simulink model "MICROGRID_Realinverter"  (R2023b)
settings: Solver=ode23tb  StartTime=0  StopTime=1.5  FixedStep=1e-3  RelTol=1e-5
undefined symbols (not defined in the file or in its folder): bridge, phase, pulses, Three
libraries: spsThreePhaseSeriesRLCBranchLib x11, simulink x10, spsThreePhaseVIMeasurementLib x9, slpidlib x8, spsMeanLib x8, spsabctodq0Lib x5, spsPLL3phLib x5, spsPower3phInstantaneousLib x5, spsRMSLib x5, spsCurrentMeasurementLib x4, spsDCVoltageSourceLib x4, spsPWMGenerator2LevelLib x4
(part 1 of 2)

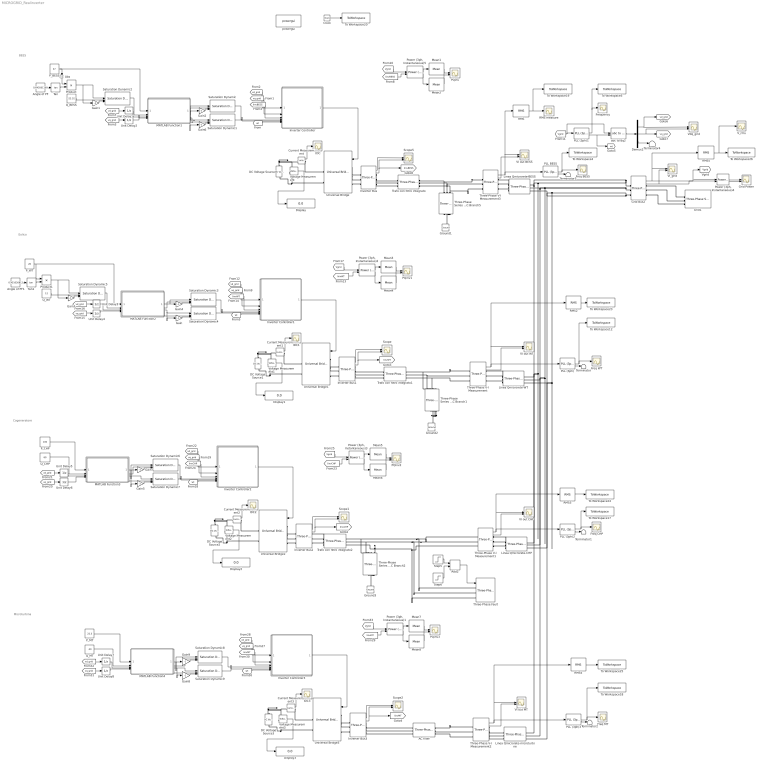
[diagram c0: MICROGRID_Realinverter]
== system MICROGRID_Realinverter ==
  note: BEES
  note: Eolico
  note: Cogeneratore
  note: Microturbina
  AC filter : spsThreePhaseSeriesRLCBranchLib/Three-Phase Series RLC Branch  LConnTagsString=A|B|C  RConnTagsString=A|B|C  BranchType=L  Resistance=0.017887  Inductance=0.536e-3  Capacitance=1e-6  Measurements=None
  Abs : Abs
  Add2 : Sum
  Angle of PF : Constant  Value=0.643501109
  Angle of PF1 : Constant  Value=0.451026812
  Clock : Clock
  Current Measurement{,1..3} (4 alike) : spsCurrentMeasurementLib/Current Measurement  PhasorSimulation=off  OutputType=Complex  PSBequivalent=0
  DC Voltage Source : spsDCVoltageSourceLib/DC Voltage Source  Amplitude=620  Measurements=None
  DC Voltage Source1 : spsDCVoltageSourceLib/DC Voltage Source  Amplitude=800  Measurements=None
  DC Voltage Source2 : spsDCVoltageSourceLib/DC Voltage Source  Amplitude=620  Measurements=None
  DC Voltage Source3 : spsDCVoltageSourceLib/DC Voltage Source  Amplitude=760  Measurements=None
  Demux2 : Demux  Outputs=3
  Display{,1..3} (4 alike) : Display
  Freq BESS : Scope
  Freq CHP : Scope
  Freq MT : Scope
  Freq WT : Scope
  Frequency : Scope
  Gain{,1..9} (10 alike) : Gain  Gain=-1
  Grid Bus2 : spsThreePhaseVIMeasurementLib/Three-Phase V-I Measurement  VoltageMeasurement=phase-to-ground  SetLabelV=off  LabelV=Vabc  Vpu=off  VpuLL=off  CurrentMeasurement=yes  SetLabelI=off  LabelI=Iabc  Ipu=off  Pbase=100e6  Vbase=500e3  OutputType=Complex  PhasorSimulation=off  PSBequivalent=0
  Grid Power : Scope  NumInputPorts=2
  Grid1 : spsThreePhaseSourceLib/Three-Phase Source  InternalConnection=Yg  VoltagePhases=off  Voltage=400  PhaseAngle=0  Voltage_phases=[25e3 25e3 25e3]/sqrt(3)  PhaseAngles_phases=[0 -120 +120]  Frequency=50  NonIdealSource=on  SpecifyImpedance=off  Resistance=86.7007e-4  Inductance=5.7558e-5  ShortCircuitLevel=100e6  BaseVoltage=400  XRratio=7  BusType=swing  Pref=10e3  Qref=0  Prefabc=[10e3, 10e3, 10e3]  Qrefabc=[0, 0, 0]  Qmin=-inf  Qmax=inf
  Ground1 : spsGroundLib/Ground  LConnTagsString=a
  Ground2 : spsGroundLib/Ground  LConnTagsString=a
  Ground3 : spsGroundLib/Ground  LConnTagsString=a
  IDC{,1..3} (4 alike) : Scope
  Inverter Controller : Subsystem  mask(Direct-Quadrature Synchronous Reference Frame Controller){Id=100, Iq=0, VDC=620, f=50, fsw=30000, L=4.388107914e-4, kp=5, ki=200}
      mask prompts: Id "Active Current (A)"; Iq "Reactive Current (A)"; VDC "DC Link Voltage (V)"; f "Grid Frequency (Hz)"; fsw "Switching Frequency (Hz)"; L "Filter Inductance (H)"; kp "Proportional Gain"; ki "Integral Gain"
      mask help: Developed by Rodney Tan (PhD) Version 1.0 (Nov 2021) This model demonstrate the operation of 3 phase grid connected inverter using Direct-Quadrature Synchronous Reference Frame Control. SPWM is use to switch the IGBT inverter bridge. The controller allows user to set the DC link voltage, active and reactive current for the inverter to be injected to the grid. The scope monitor the grid inverter output voltage and current waveform. The display monitor the active and reactive power injected to the grid.
  Inverter Controller1 : Subsystem  mask(Direct-Quadrature Synchronous Reference Frame Controller){Id=100, Iq=0, VDC=800, f=50, fsw=30000, L=9.11597e-4, kp=1.3, ki=25}
      mask prompts: Id "Active Current (A)"; Iq "Reactive Current (A)"; VDC "DC Link Voltage (V)"; f "Grid Frequency (Hz)"; fsw "Switching Frequency (Hz)"; L "Filter Inductance (H)"; kp "Proportional Gain"; ki "Integral Gain"
      mask help: Developed by Rodney Tan (PhD) Version 1.0 (Nov 2021) This model demonstrate the operation of 3 phase grid connected inverter using Direct-Quadrature Synchronous Reference Frame Control. SPWM is use to switch the IGBT inverter bridge. The controller allows user to set the DC link voltage, active and reactive current for the inverter to be injected to the grid. The scope monitor the grid inverter output voltage and current waveform. The display monitor the active and reactive power injected to the grid.
  Inverter Controller2 : Subsystem  mask(Direct-Quadrature Synchronous Reference Frame Controller){Id=100, Iq=0, VDC=620, f=50, fsw=30000, L=10.3395525582e-4, kp=2.5, ki=100}
      mask prompts: Id "Active Current (A)"; Iq "Reactive Current (A)"; VDC "DC Link Voltage (V)"; f "Grid Frequency (Hz)"; fsw "Switching Frequency (Hz)"; L "Filter Inductance (H)"; kp "Proportional Gain"; ki "Integral Gain"
      mask help: Developed by Rodney Tan (PhD) Version 1.0 (Nov 2021) This model demonstrate the operation of 3 phase grid connected inverter using Direct-Quadrature Synchronous Reference Frame Control. SPWM is use to switch the IGBT inverter bridge. The controller allows user to set the DC link voltage, active and reactive current for the inverter to be injected to the grid. The scope monitor the grid inverter output voltage and current waveform. The display monitor the active and reactive power injected to the grid.
  Inverter Controller3 : Subsystem  mask(Direct-Quadrature Synchronous Reference Frame Controller){Id=100, Iq=0, VDC=760, f=50, fsw=30000, L=0.55535e-3, kp=10, ki=20}
      mask prompts: Id "Active Current (A)"; Iq "Reactive Current (A)"; VDC "DC Link Voltage (V)"; f "Grid Frequency (Hz)"; fsw "Switching Frequency (Hz)"; L "Filter Inductance (H)"; kp "Proportional Gain"; ki "Integral Gain"
      mask help: Developed by Rodney Tan (PhD) Version 1.0 (Nov 2021) This model demonstrate the operation of 3 phase grid connected inverter using Direct-Quadrature Synchronous Reference Frame Control. SPWM is use to switch the IGBT inverter bridge. The controller allows user to set the DC link voltage, active and reactive current for the inverter to be injected to the grid. The scope monitor the grid inverter output voltage and current waveform. The display monitor the active and reactive power injected to the grid.
  Inverter Bus{,1..3} (4 alike) : spsThreePhaseVIMeasurementLib/Three-Phase V-I Measurement  VoltageMeasurement=phase-to-ground  SetLabelV=off  LabelV=Vabc  Vpu=off  VpuLL=off  CurrentMeasurement=yes  SetLabelI=off  LabelI=Iabc  Ipu=off  Pbase=100e6  Vbase=500e3  OutputType=Complex  PhasorSimulation=off  PSBequivalent=0
  Linea Qmicrorete-BESS : spsThreePhaseSeriesRLCBranchLib/Three-Phase Series RLC Branch  LConnTagsString=A|B|C  RConnTagsString=A|B|C  BranchType=RL  Resistance=0.03105  Inductance=3.111479137e-5  Capacitance=1e-6  Measurements=None
  Linea Qmicrorete-CHP : spsThreePhaseSeriesRLCBranchLib/Three-Phase Series RLC Branch  LConnTagsString=A|B|C  RConnTagsString=A|B|C  BranchType=RL  Resistance=0.01092  Inductance=2.7072255e-5  Capacitance=1e-6  Measurements=None
  Linea Qmicrorete-WT : spsThreePhaseSeriesRLCBranchLib/Three-Phase Series RLC Branch  LConnTagsString=A|B|C  RConnTagsString=A|B|C  BranchType=RL  Resistance=0.0071  Inductance=2.89661996e-6  Capacitance=1e-6  Measurements=None
  Linea Qmicrorete-microturbine : spsThreePhaseSeriesRLCBranchLib/Three-Phase Series RLC Branch  LConnTagsString=A|B|C  RConnTagsString=A|B|C  BranchType=RL  Resistance=0.0852  Inductance=2.826591789e-5  Capacitance=1e-6  Measurements=None
  MATLAB Function1 : MATLAB Function  TreatAsAtomicUnit=on
  MATLAB Function2 : MATLAB Function  TreatAsAtomicUnit=on
  MATLAB Function3 : MATLAB Function  TreatAsAtomicUnit=on
  MATLAB Function4 : MATLAB Function  TreatAsAtomicUnit=on
  Mean{1..8} (8 alike) : spsMeanLib/Mean  Freq=50  Vinit=0  Ts=0
  PLL (3ph) : spsPLL3phLib/PLL (3ph)  Fmin=45  Par_Init=[0, 60]  ParK=[180, 3200, 1]  TcD=1e-4  MaxRateChangeFreq=12  FilterCutOffFreq=25  Ts=0  AGC=on
  PLL (3ph)1 : spsPLL3phLib/PLL (3ph)  Fmin=45  Par_Init=[0, 50]  ParK=[180, 3200, 1]  TcD=1e-4  MaxRateChangeFreq=12  FilterCutOffFreq=25  Ts=0  AGC=on
  PLL (3ph)2 : spsPLL3phLib/PLL (3ph)  Fmin=45  Par_Init=[0, 60]  ParK=[180, 3200, 1]  TcD=1e-4  MaxRateChangeFreq=12  FilterCutOffFreq=25  Ts=0  AGC=on
  PLL (3ph)3 : spsPLL3phLib/PLL (3ph)  Fmin=45  Par_Init=[0, 60]  ParK=[180, 3200, 1]  TcD=1e-4  MaxRateChangeFreq=12  FilterCutOffFreq=25  Ts=0  AGC=on
  PLL BESS : spsPLL3phLib/PLL (3ph)  Fmin=45  Par_Init=[0, 60]  ParK=[180, 3200, 1]  TcD=1e-4  MaxRateChangeFreq=12  FilterCutOffFreq=25  Ts=0  AGC=on
  PQinv{,1..3} (4 alike) : Scope  NumInputPorts=2
  P_BESS : Constant  Value=37
  P_CHP : Constant  Value=100
  P_MT : Constant  Value=22.3
  P_WT : Constant  Value=26
  Power (3ph, Instantaneous){1..5} (5 alike) : spsPower3phInstantaneousLib/Power (3ph, Instantaneous)
  Product : Product
  Product1 : Product
  Q_BESS : Constant  Value=-22.32
  Q_CHP : Constant  Value=60
  Q_MT : Constant  Value=-30
  Q_WT : Constant  Value=12
  RMS{,2..5} (5 alike) : spsRMSLib/RMS  TrueRMS=on  Freq=50  RMSInit=0  Ts=0
  RMS measure : Scope
  Saturation Dynamic{,1..9} (10 alike) : simulink/Discontinuities/Saturation Dynamic  OutMin=[]  OutMax=[]  OutDataTypeStr=Inherit: Same as second input  OutDataType=fixdt(1, 16)  OutScaling=2^-10  DoSatur=off
  Scope{,1..2,5} (4 alike) : Scope  NumInputPorts=2
  Step5 : Step  Time=1.1
  Step6 : Step  Time=1.2  After=-1
  Tan : Trigonometry  Operator=tan
  Tan1 : Trigonometry  Operator=tan
  Terminator{,1..4} (5 alike) : Terminator
  Three-Phase Series RLC Branch1 : spsThreePhaseSeriesRLCBranchLib/Three-Phase Series RLC Branch  LConnTagsString=A|B|C  RConnTagsString=A|B|C  BranchType=C  Resistance=1  Inductance=1e-3  Capacitance=8.33333333333333333333333333e-6  Measurements=None
  Three-Phase Series RLC Branch2 : spsThreePhaseSeriesRLCBranchLib/Three-Phase Series RLC Branch  LConnTagsString=A|B|C  RConnTagsString=A|B|C  BranchType=C  Resistance=1  Inductance=1e-3  Capacitance=800e-6  Measurements=None
  Three-Phase Series RLC Branch5 : spsThreePhaseSeriesRLCBranchLib/Three-Phase Series RLC Branch  LConnTagsString=A|B|C  RConnTagsString=A|B|C  BranchType=C  Resistance=1  Inductance=1e-3  Capacitance=1.7954e-4  Measurements=None
  Three-Phase V-I Measurement{,1..3} (4 alike) : spsThreePhaseVIMeasurementLib/Three-Phase V-I Measurement  VoltageMeasurement=phase-to-ground  SetLabelV=off  LabelV=Vabc  Vpu=off  VpuLL=off  CurrentMeasurement=yes  SetLabelI=off  LabelI=Iabc  Ipu=off  Pbase=100e6  Vbase=500e3  OutputType=Complex  PhasorSimulation=off  PSBequivalent=0
  Three-Phase Fault : spsThreePhaseFaultLib/Three-Phase Fault  InitialStates=0  FaultA=on  FaultB=on  FaultC=on  GroundFault=off  SwitchTimes="[1/60  5/60]"  External=on  SwitchStatus=NaN  FaultResistance=0.06  GroundResistance=0.01  SnubberResistance=1e6  SnubberCapacitance=0  Measurements=None
  To Workspace12 : ToWorkspace  VariableName=Freq_WT  SampleTime=0.02
  To Workspace17 : ToWorkspace  VariableName=Freq_CHP  SampleTime=0.02
  To Workspace18 : ToWorkspace  VariableName=Freq_Mt  SampleTime=0.02
  To Workspace19 : ToWorkspace  VariableName=V_out_BESS_rms  SampleTime=0.02
  To Workspace20 : ToWorkspace  VariableName=time  SampleTime=0.02
  To Workspace23 : ToWorkspace  VariableName=V_out_WT_rms  SampleTime=0.02
  To Workspace24 : ToWorkspace  VariableName=V_out_CHP_rms  SampleTime=0.02
  To Workspace25 : ToWorkspace  VariableName=V_inv_MT_rms  SampleTime=0.02
  To Workspace26 : ToWorkspace  VariableName=V_out_Grid_rms  SampleTime=0.02
  To Workspace4 : ToWorkspace  VariableName=Freq_BESS  SampleTime=0.02
  To Workspace5 : ToWorkspace  VariableName=Freq_Grid  SampleTime=0.02
  Trafo con filtro integrato : spsThreePhaseSeriesRLCBranchLib/Three-Phase Series RLC Branch  LConnTagsString=A|B|C  RConnTagsString=A|B|C  BranchType=RL  Resistance=0.04996  Inductance=4.07696e-4  Capacitance=1e-6  Measurements=None
  Trafo con filtro integrato1 : spsThreePhaseSeriesRLCBranchLib/Three-Phase Series RLC Branch  LConnTagsString=A|B|C  RConnTagsString=A|B|C  BranchType=RL  Resistance=0.0362  Inductance=9.087e-4  Capacitance=1e-6  Measurements=None
  Trafo con filtro integrato2 : spsThreePhaseSeriesRLCBranchLib/Three-Phase Series RLC Branch  LConnTagsString=A|B|C  RConnTagsString=A|B|C  BranchType=RL  Resistance=0.017887  Inductance=10.06883e-4  Capacitance=1e-6  Measurements=None
  Unit Delay{1..8} (8 alike) : UnitDelay  InitialCondition=0.01  SampleTime=-1  HasFrameUpgradeWarning=on
  Universal Bridge{,1..3} (4 alike) : spsUniversalBridgeLib/Universal Bridge  Arms=3  SnubberResistance=1e5  SnubberCapacitance=inf  Device=IGBT / Diodes  Ron=1e-3  Lon=0  ForwardVoltages="[  0  0  ]"  ForwardVoltage=0  GTOparameters=[ 10e-6 , 20e-6 ]  IGBTparameters=[ 1e-6 , 2e-6 ]  Measurements=None  Measurements_2=None  converterType=Rectifier
  VI out BESS : Scope  NumInputPorts=2
  VI out CHP : Scope  NumInputPorts=2
  VI out MT : Scope  NumInputPorts=2
  VI out WT : Scope  NumInputPorts=2
  VI_grid : Scope  NumInputPorts=2
  V_rms : Scope
  Vdq_grid : Scope  NumInputPorts=2
  Voltage Measurement{,1..3} (4 alike) : spsVoltageMeasurementLib/Voltage Measurement  PhasorSimulation=off  OutputType=Complex  PSBequivalent=0
  abc to dq2 : spsabctodq0Lib/abc to dq0  Alignment=90 degrees behind phase A axis
  powergui : spspowerguiLib/powergui  Priority=1  SimulationMode=Discrete  SampleTime=1e-6  frequency=60  Iterations=50  frequencyindice=0  Pbase=100e6  ErrMax=1e-4  UnitsV=kV  UnitsW=MW  buscounter=0  FunctionMessages=off  echomessages=off  EnableUseOfTLC=off  CurrentSourceSwitches=off  DisableSnubberDevices=off  DisableRonSwitches=off  DisableVfSwitches=off  DisplayEquations=off  AutomaticDiscreteSolvers=off  SolverType=Tustin/Backward Euler (TBE)  Interpol=off  ExternalGateDelay=off  methode=off  Ts=100  x0status=blocks  SPID=on  SwTol=0  HookPort=off  NonlinearTolerance=1e-4  nMaxIteration=100  ContinueOnMaxIteration=off  RestoreLinks=warning  ResistiveCurrentMeasurement=off  Frange=[0:2:500]  Ylog=off  Xlog=on  ShowGrid=off  save=off  variable=ZData  structure=0  ZoomFFT=off  StartTime=0.0  cycles=1  DisplayStyle=1  fundamental=60  FreqAxis=off  MaxFrequency=1000  frequencyindicesteady=1  RmsSteady=1  display=off
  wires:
  Demux2/3 -> Terminator4/1
  Demux2/2 -> Vdq_grid/2, [vq_grid]
  [Vgrid] -> abc to dq2/1, PLL (3ph)1/1
  PLL (3ph)1/2 -> [wt], abc to dq2/2
  Grid Bus2/2 -> "Power (3ph, Instantaneous)4"/2, VI_grid/2
  Grid Bus2/1 -> [Vgrid], "Power (3ph, Instantaneous)4"/1, RMS5/1, VI_grid/1
  PLL (3ph)1/1 -> To Workspace5/1, Frequency/1
  Demux2/1 -> [vd_grid], Vdq_grid/1
  abc to dq2/1 -> Demux2/1
  Three-Phase V-I Measurement/1 -> PLL (3ph)/1, VI out WT/1, RMS2/1
  PLL (3ph)/1 -> Freq WT/1, To Workspace12/1
  Three-Phase V-I Measurement/2 -> VI out WT/2
  PLL (3ph)2/1 -> Freq CHP/1, To Workspace17/1
  PLL (3ph)3/1 -> To Workspace18/1, Freq MT/1
  PLL (3ph)/2 -> Terminator/1
  PLL (3ph)2/2 -> Terminator1/1
  PLL (3ph)3/2 -> Terminator2/1
  Three-Phase V-I Measurement3/1 -> PLL BESS/1, RMS/1, VI out BESS/1
  PLL BESS/1 -> Freq BESS/1, To Workspace4/1
  Three-Phase V-I Measurement3/2 -> VI out BESS/2
  PLL BESS/2 -> Terminator3/1
  "Power (3ph, Instantaneous)4"/1 -> Grid Power/1
  "Power (3ph, Instantaneous)4"/2 -> Grid Power/2
  Three-Phase V-I Measurement1/1 -> PLL (3ph)2/1, RMS3/1, VI out CHP/1
  Three-Phase V-I Measurement1/2 -> VI out CHP/2
  Three-Phase V-I Measurement2/2 -> VI out MT/2
  Three-Phase V-I Measurement2/1 -> PLL (3ph)3/1, RMS4/1, VI out MT/1
  RMS/1 -> To Workspace19/1, RMS measure/1
  RMS2/1 -> To Workspace23/1
  RMS3/1 -> To Workspace24/1
  RMS4/1 -> To Workspace25/1
  RMS5/1 -> V_rms/1, To Workspace26/1
  Clock/1 -> To Workspace20/1
  Saturation Dynamic1/1 -> Inverter Controller/5(Iq*)
  Inverter Controller/1(PWM) -> Universal Bridge/1
  Angle of PF/1 -> Tan/1
  P_BESS/1 -> MATLAB Function1/1(Pe), Abs/1
  [vd_grid] -> Unit Delay1/1
  Tan/1 -> Product/2
  MATLAB Function1/4(Iq) -> Saturation Dynamic1/2
  MATLAB Function1/2(Id) -> Saturation Dynamic/2
  Gain1/1 -> Saturation Dynamic2/3
  Gain2/1 -> Saturation Dynamic/3
  MATLAB Function1/1(Id1) -> Saturation Dynamic/1, Gain2/1
  Saturation Dynamic2/1 -> MATLAB Function1/2(Qe)
  MATLAB Function1/3(Iq1) -> Gain6/1, Saturation Dynamic1/1
  [vq_grid] -> Unit Delay2/1
  Abs/1 -> Product/1
  [IinvBESS] -> Inverter Controller/3(Iinv)
  Unit Delay1/1 -> MATLAB Function1/3(Vd_grid)
  Inverter Bus/2 -> [IinvBESS], Scope5/2
  Product/1 -> Gain1/1, Saturation Dynamic2/1
  Voltage Measurement/1 -> Display/1
  [vd_grid] -> Inverter Controller/1(vd_grid)
  [vq_grid] -> Inverter Controller/2(vq_grid)
  Q_BESS/1 -> Saturation Dynamic2/2
  Saturation Dynamic/1 -> Inverter Controller/4(id*)
  Gain6/1 -> Saturation Dynamic1/3
  Current Measurement/1 -> IDC/1
  Inverter Bus/1 -> Scope5/1
  [wt] -> Inverter Controller/6(wt)
  Unit Delay2/1 -> MATLAB Function1/4(Vq_grid)
  Mean1/1 -> PQinv/1
  "Power (3ph, Instantaneous)5"/1 -> Mean1/1
  "Power (3ph, Instantaneous)5"/2 -> Mean2/1
  [IinvBESS] -> "Power (3ph, Instantaneous)5"/2
  Mean2/1 -> PQinv/2
  [Vgrid] -> "Power (3ph, Instantaneous)5"/1
  MATLAB Function2/3(Iq1) -> Gain/1, Saturation Dynamic4/1
  Tan1/1 -> Product1/2
  [IinvWT] -> Inverter Controller1/3(Iinv)
  Saturation Dynamic4/1 -> Inverter Controller1/5(Iq*)
  Saturation Dynamic3/1 -> Inverter Controller1/4(id*)
  "Power (3ph, Instantaneous)2"/1 -> Mean3/1
  Current Measurement1/1 -> IDC1/1
  MATLAB Function2/4(Iq) -> Saturation Dynamic4/2
  [vq_grid] -> Unit Delay4/1
  Unit Delay4/1 -> MATLAB Function2/4(Vq_grid)
  Gain3/1 -> Saturation Dynamic5/3
  Product1/1 -> Gain3/1, Saturation Dynamic5/1
  Mean3/1 -> PQinv1/1
  Inverter Bus1/1 -> Scope/1
  Unit Delay3/1 -> MATLAB Function2/3(Vd_grid)
  [wt] -> Inverter Controller1/6(wt)
  [vd_grid] -> Inverter Controller1/1(vd_grid)
  Inverter Controller1/1(PWM) -> Universal Bridge1/1
  Voltage Measurement1/1 -> Display1/1
  "Power (3ph, Instantaneous)2"/2 -> Mean4/1
  [vq_grid] -> Inverter Controller1/2(vq_grid)
  Saturation Dynamic5/1 -> MATLAB Function2/2(Qe)
  [IinvWT] -> "Power (3ph, Instantaneous)2"/2
  P_WT/1 -> MATLAB Function2/1(Pe), Product1/1
  Mean4/1 -> PQinv1/2
  Angle of PF1/1 -> Tan1/1
  Gain4/1 -> Saturation Dynamic3/3
  Q_WT/1 -> Saturation Dynamic5/2
  Inverter Bus1/2 -> [IinvWT], Scope/2
  MATLAB Function2/2(Id) -> Saturation Dynamic3/2
  MATLAB Function2/1(Id1) -> Gain4/1, Saturation Dynamic3/1
  [vd_grid] -> Unit Delay3/1
  Gain/1 -> Saturation Dynamic4/3
  [Vgrid] -> "Power (3ph, Instantaneous)2"/1
  Saturation Dynamic7/1 -> Inverter Controller2/5(Iq*)
  Mean6/1 -> PQinv2/2
  [vq_grid] -> Unit Delay6/1
  Mean5/1 -> PQinv2/1
  [IinvCHP] -> Inverter Controller2/3(Iinv)
  Voltage Measurement2/1 -> Display2/1
  MATLAB Function3/3(Iq1) -> Gain5/1, Saturation Dynamic7/1
  MATLAB Function3/1(Id1) -> Gain7/1, Saturation Dynamic6/1
  Saturation Dynamic6/1 -> Inverter Controller2/4(id*)
  [vd_grid] -> Unit Delay5/1
  P_CHP/1 -> MATLAB Function3/1(Pe)
  Gain5/1 -> Saturation Dynamic7/3
  Q_CHP/1 -> MATLAB Function3/2(Qe)
  "Power (3ph, Instantaneous)3"/2 -> Mean6/1
  Unit Delay5/1 -> MATLAB Function3/3(Vd_grid)
  MATLAB Function3/4(Iq) -> Saturation Dynamic7/2
  Inverter Bus2/1 -> Scope1/1
  Unit Delay6/1 -> MATLAB Function3/4(Vq_grid)
  [IinvCHP] -> "Power (3ph, Instantaneous)3"/2
  Inverter Controller2/1(PWM) -> Universal Bridge2/1
  "Power (3ph, Instantaneous)3"/1 -> Mean5/1
  MATLAB Function3/2(Id) -> Saturation Dynamic6/2
  [wt] -> Inverter Controller2/6(wt)
  Gain7/1 -> Saturation Dynamic6/3
  [vd_grid] -> Inverter Controller2/1(vd_grid)
  Inverter Bus2/2 -> [IinvCHP], Scope1/2
  Current Measurement2/1 -> IDC2/1
  [vq_grid] -> Inverter Controller2/2(vq_grid)
  [Vgrid] -> "Power (3ph, Instantaneous)3"/1
  MATLAB Function4/2(Id) -> Saturation Dynamic8/2
  Current Measurement3/1 -> IDC3/1
  Gain9/1 -> Saturation Dynamic8/3
  P_MT/1 -> MATLAB Function4/1(Pe)
  Unit Delay8/1 -> MATLAB Function4/4(Vq_grid)
  [IinvMT] -> "Power (3ph, Instantaneous)1"/2
  Unit Delay7/1 -> MATLAB Function4/3(Vd_grid)
  MATLAB Function4/4(Iq) -> Saturation Dynamic9/2
  [vq_grid] -> Unit Delay8/1
  [IinvMT] -> Inverter Controller3/3(Iinv)
  Inverter Bus3/1 -> Scope2/1
  Q_MT/1 -> MATLAB Function4/2(Qe)
  Inverter Bus3/2 -> [IinvMT], Scope2/2
  [wt] -> Inverter Controller3/6(wt)
  MATLAB Function4/3(Iq1) -> Gain8/1, Saturation Dynamic9/1
  [vd_grid] -> Unit Delay7/1
  Gain8/1 -> Saturation Dynamic9/3
  Saturation Dynamic8/1 -> Inverter Controller3/4(id*)
  Inverter Controller3/1(PWM) -> Universal Bridge3/1
  Mean7/1 -> PQinv3/1
  MATLAB Function4/1(Id1) -> Gain9/1, Saturation Dynamic8/1
  Saturation Dynamic9/1 -> Inverter Controller3/5(Iq*)
  "Power (3ph, Instantaneous)1"/2 -> Mean8/1
  "Power (3ph, Instantaneous)1"/1 -> Mean7/1
  [vq_grid] -> Inverter Controller3/2(vq_grid)
  Mean8/1 -> PQinv3/2
  [vd_grid] -> Inverter Controller3/1(vd_grid)
  Voltage Measurement3/1 -> Display3/1
  Step5/1 -> Add2/1
  Step6/1 -> Add2/2
  Add2/1 -> Three-Phase Fault/1
  [Vgrid] -> "Power (3ph, Instantaneous)1"/1
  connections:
  Grid1/RConn2 -- Grid Bus2/RConn2
  Grid1/RConn3 -- Grid Bus2/RConn3
  Grid1/RConn1 -- Grid Bus2/RConn1
  Grid Bus2/LConn3 -- Linea Qmicrorete-WT/RConn3 -- Linea Qmicrorete-microturbine/RConn3 -- Linea Qmicrorete-CHP/RConn3 -- Linea Qmicrorete-BESS/RConn3
  Grid Bus2/LConn2 -- Linea Qmicrorete-WT/RConn2 -- Linea Qmicrorete-microturbine/RConn2 -- Linea Qmicrorete-CHP/RConn2 -- Linea Qmicrorete-BESS/RConn2
  Grid Bus2/LConn1 -- Linea Qmicrorete-WT/RConn1 -- Linea Qmicrorete-microturbine/RConn1 -- Linea Qmicrorete-CHP/RConn1 -- Linea Qmicrorete-BESS/RConn1
  Linea Qmicrorete-CHP/LConn1 -- Three-Phase V-I Measurement1/RConn1
  Linea Qmicrorete-CHP/LConn2 -- Three-Phase V-I Measurement1/RConn2
  Linea Qmicrorete-CHP/LConn3 -- Three-Phase V-I Measurement1/RConn3
  Three-Phase V-I Measurement2/RConn1 -- Linea Qmicrorete-microturbine/LConn1
  Three-Phase V-I Measurement2/RConn2 -- Linea Qmicrorete-microturbine/LConn2
  Three-Phase V-I Measurement2/RConn3 -- Linea Qmicrorete-microturbine/LConn3
  Linea Qmicrorete-BESS/LConn1 -- Three-Phase V-I Measurement3/RConn1
  Linea Qmicrorete-BESS/LConn2 -- Three-Phase V-I Measurement3/RConn2
  Linea Qmicrorete-BESS/LConn3 -- Three-Phase V-I Measurement3/RConn3
  Linea Qmicrorete-WT/LConn1 -- Three-Phase V-I Measurement/RConn1
  Linea Qmicrorete-WT/LConn2 -- Three-Phase V-I Measurement/RConn2
  Linea Qmicrorete-WT/LConn3 -- Three-Phase V-I Measurement/RConn3
  Three-Phase Series RLC Branch5/LConn3 -- Three-Phase V-I Measurement3/LConn3 -- Trafo con filtro integrato/RConn3
  Three-Phase Series RLC Branch5/LConn1 -- Three-Phase V-I Measurement3/LConn1 -- Trafo con filtro integrato/RConn1
  Three-Phase Series RLC Branch5/RConn1 -- Three-Phase Series RLC Branch5/RConn2 -- Three-Phase Series RLC Branch5/RConn3 -- Ground1/LConn1
  Three-Phase Series RLC Branch5/LConn2 -- Three-Phase V-I Measurement3/LConn2 -- Trafo con filtro integrato/RConn2
  Voltage Measurement/LConn2 -- DC Voltage Source/LConn1 -- Universal Bridge/RConn2
  DC Voltage Source/RConn1 -- Current Measurement/LConn1 -- Voltage Measurement/LConn1
  Universal Bridge/LConn2 -- Inverter Bus/LConn2
  Universal Bridge/LConn3 -- Inverter Bus/LConn3
  Current Measurement/RConn1 -- Universal Bridge/RConn1
  Universal Bridge/LConn1 -- Inverter Bus/LConn1
  Inverter Bus/RConn2 -- Trafo con filtro integrato/LConn2
  Inverter Bus/RConn1 -- Trafo con filtro integrato/LConn1
  Inverter Bus/RConn3 -- Trafo con filtro integrato/LConn3
  Trafo con filtro integrato1/RConn2 -- Three-Phase V-I Measurement/LConn2 -- Three-Phase Series RLC Branch1/LConn2
  DC Voltage Source1/RConn1 -- Current Measurement1/LConn1 -- Voltage Measurement1/LConn1
  Voltage Measurement1/LConn2 -- DC Voltage Source1/LConn1 -- Universal Bridge1/RConn2
  Three-Phase Series RLC Branch1/RConn3 -- Three-Phase Series RLC Branch1/RConn2 -- Ground2/LConn1 -- Three-Phase Series RLC Branch1/RConn1
  Trafo con filtro integrato1/RConn1 -- Three-Phase V-I Measurement/LConn1 -- Three-Phase Series RLC Branch1/LConn1
  Trafo con filtro integrato1/RConn3 -- Three-Phase V-I Measurement/LConn3 -- Three-Phase Series RLC Branch1/LConn3
  Inverter Bus1/RConn3 -- Trafo con filtro integrato1/LConn3
  Inverter Bus1/RConn2 -- Trafo con filtro integrato1/LConn2
  Universal Bridge1/LConn2 -- Inverter Bus1/LConn2
  Current Measurement1/RConn1 -- Universal Bridge1/RConn1
  Universal Bridge1/LConn1 -- Inverter Bus1/LConn1
  Inverter Bus1/RConn1 -- Trafo con filtro integrato1/LConn1
  Universal Bridge1/LConn3 -- Inverter Bus1/LConn3
  Three-Phase Series RLC Branch2/LConn3 -- Three-Phase Fault/LConn3 -- Three-Phase V-I Measurement1/LConn3 -- Trafo con filtro integrato2/RConn3
  DC Voltage Source2/RConn1 -- Current Measurement2/LConn1 -- Voltage Measurement2/LConn1
  Trafo con filtro integrato2/RConn2 -- Three-Phase V-I Measurement1/LConn2 -- Three-Phase Fault/LConn2 -- Three-Phase Series RLC Branch2/LConn2
  Three-Phase Series RLC Branch2/RConn1 -- Three-Phase Series RLC Branch2/RConn2 -- Three-Phase Series RLC Branch2/RConn3 -- Ground3/LConn1
  Trafo con filtro integrato2/RConn1 -- Three-Phase V-I Measurement1/LConn1 -- Three-Phase Fault/LConn1 -- Three-Phase Series RLC Branch2/LConn1
  Voltage Measurement2/LConn2 -- DC Voltage Source2/LConn1 -- Universal Bridge2/RConn2
  Trafo con filtro integrato2/LConn2 -- Inverter Bus2/RConn2
  Universal Bridge2/LConn3 -- Inverter Bus2/LConn3
  Universal Bridge2/LConn1 -- Inverter Bus2/LConn1
  Current Measurement2/RConn1 -- Universal Bridge2/RConn1
  Trafo con filtro integrato2/LConn3 -- Inverter Bus2/RConn3
  Universal Bridge2/LConn2 -- Inverter Bus2/LConn2
  Trafo con filtro integrato2/LConn1 -- Inverter Bus2/RConn1
  DC Voltage Source3/RConn1 -- Current Measurement3/LConn1 -- Voltage Measurement3/LConn1
  Voltage Measurement3/LConn2 -- DC Voltage Source3/LConn1 -- Universal Bridge3/RConn2
  Inverter Bus3/RConn3 -- AC filter/LConn3
  Universal Bridge3/LConn3 -- Inverter Bus3/LConn3
  AC filter/RConn3 -- Three-Phase V-I Measurement2/LConn3
  AC filter/RConn1 -- Three-Phase V-I Measurement2/LConn1
  AC filter/RConn2 -- Three-Phase V-I Measurement2/LConn2
  Universal Bridge3/LConn2 -- Inverter Bus3/LConn2
  Inverter Bus3/RConn2 -- AC filter/LConn2
  Current Measurement3/RConn1 -- Universal Bridge3/RConn1
  Universal Bridge3/LConn1 -- Inverter Bus3/LConn1
  Inverter Bus3/RConn1 -- AC filter/LConn1

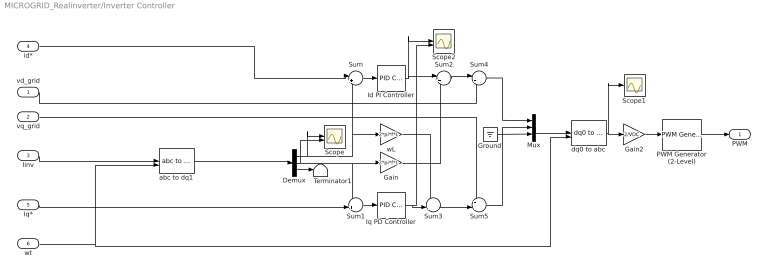
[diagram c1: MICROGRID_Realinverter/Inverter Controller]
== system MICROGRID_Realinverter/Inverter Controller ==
  vd_grid : Inport
  vq_grid : Inport  Port=2
  Iinv : Inport  Port=3
  id* : Inport  Port=4
  Iq* : Inport  Port=5
  wt : Inport  Port=6
  Demux : Demux  Outputs=3
  Gain : Gain  Gain=2*pi*f*L
  Gain2 : Gain  Gain=2/VDC
  Ground : Ground
  Id PI Controller : slpidlib/PID Controller  Controller=PI  Form=Parallel  TimeDomain=Continuous-time  UseExternalTs=off  SampleTime=-1  IntegratorMethod=Forward Euler  FilterMethod=Forward Euler  ControllerParametersSource=internal  P=kp  I=ki  UseKiTs=off  D=0  N=100  UseFilter=on  TunerSelectOption=Transfer Function Based (PID Tuner App)  InitialConditionSource=internal  InitialConditionForIntegrator=0  InitialConditionForFilter=0  DifferentiatorICPrevScaledInput=0  ExternalReset=none  TrackingMode=off  Kt=1  LimitOutput=off  SatLimitsSource=internal  UpperSaturationLimit=inf  LowerSaturationLimit=-inf  LinearizeAsGain=on  AntiWindupMode=none  Kb=1  LimitIntegrator=off  UpperIntegratorSaturationLimit=inf  LowerIntegratorSaturationLimit=-inf  POutMin=[]  POutMax=[]  IOutMin=[]  IOutMax=[]  DOutMin=[]  DOutMax=[]  NOutMin=[]  NOutMax=[]  SumOutMin=[]  SumOutMax=[]  SaturationOutMin=[]  SaturationOutMax=[]  PParamMin=[]  PParamMax=[]  IParamMin=[]  IParamMax=[]  DParamMin=[]  DParamMax=[]  NParamMin=[]  NParamMax=[]  KbParamMin=[]  KbParamMax=[]  KtParamMin=[]  KtParamMax=[]  KbOutMin=[]  KbOutMax=[]  KtOutMin=[]  KtOutMax=[]  IntegratorOutMin=[]  IntegratorOutMax=[]  FilterOutMin=[]  FilterOutMax=[]  SumI1OutMin=[]  SumI1OutMax=[]  SumI2OutMin=[]  SumI2OutMax=[]  SumI3OutMin=[]  SumI3OutMax=[]  SumI4OutMin=[]  SumI4OutMax=[]  SumDOutMin=[]  SumDOutMax=[]  DifferentiatorOutMin=[]  DifferentiatorOutMax=[]  FilterDiffOutCoefMin=[]  FilterDiffOutCoefMax=[]  ReciprocalOutMin=[]  ReciprocalOutMax=[]  SumDenOutMin=[]  SumDenOutMax=[]  SumNumOutMin=[]  SumNumOutMax=[]  DivideOutMin=[]  DivideOutMax=[]  UdiffTsProdOutMin=[]  UdiffTsProdOutMax=[]  NTsProdOutMin=[]  NTsProdOutMax=[]  UintegralTsProdOutMin=[]  UintegralTsProdOutMax=[]  UngainTsProdOutMin=[]  UngainTsProdOutMax=[]  ClampingZeroOutDataTypeStr=Inherit: Inherit via back propagation  ClampingZeroOutMin=[]  ClampingZeroOutMax=[]  FilterDenConstantOutDataTypeStr=Inherit: Inherit via back propagation  FilterDenConstantOutMin=[]  FilterDenConstantOutMax=[]  PCopyOutDataTypeStr=Inherit: Inherit via back propagation  PCopyOutMin=[]  PCopyOutMax=[]  NCopyOutDataTypeStr=Inherit: Inherit via back propagation  NCopyOutMin=[]  NCopyOutMax=[]  IntegratorContinuousStateAttributes=''  IntegratorStateMustResolveToSignalObject=off  IntegratorRTWStateStorageClass=Auto  FilterContinuousStateAttributes=''  FilterStateMustResolveToSignalObject=off  FilterRTWStateStorageClass=Auto  ParallelPVariant=InternalParameters  IdealPVariant=Disabled  IVariant=InternalParameters  DVariant=Disabled  IntegratorVariant=Continuous  SatVariant=Disabled  AWVariant=Passthrough  PCopyVariant=Disabled  TRVariant=Disabled  FdbkBlocksVariant=Forward  IdealPFdbkVariant=Disabled  SatFdbkVariant=Disabled  DerivativeFilterVariant=Disabled  NVariant=Disabled  NCopyVariant=Disabled_SignalSpec  FilterICVariant=Disabled  IntegratorICVariant=InternalICs  ExternalResetVariant=Disabled  TRSumVariant=Passthrough  SumFdbkVariant=Disabled  SumVariant=Sum_PI  TsampFilterVariant=InternalTs  TsampNgainVariant=Passthrough  TsampIntegralVariant=Disabled_SignalSpec  ExternalSaturationOutDataTypeStr=Inherit: Same as second input
  Iq PD Controller : slpidlib/PID Controller  Controller=PI  Form=Parallel  TimeDomain=Continuous-time  UseExternalTs=off  SampleTime=-1  IntegratorMethod=Forward Euler  FilterMethod=Forward Euler  ControllerParametersSource=internal  P=kp  I=ki  UseKiTs=off  D=0  N=100  UseFilter=on  TunerSelectOption=Transfer Function Based (PID Tuner App)  InitialConditionSource=internal  InitialConditionForIntegrator=0  InitialConditionForFilter=0  DifferentiatorICPrevScaledInput=0  ExternalReset=none  TrackingMode=off  Kt=1  LimitOutput=off  SatLimitsSource=internal  UpperSaturationLimit=inf  LowerSaturationLimit=-inf  LinearizeAsGain=on  AntiWindupMode=none  Kb=1  LimitIntegrator=off  UpperIntegratorSaturationLimit=inf  LowerIntegratorSaturationLimit=-inf  POutMin=[]  POutMax=[]  IOutMin=[]  IOutMax=[]  DOutMin=[]  DOutMax=[]  NOutMin=[]  NOutMax=[]  SumOutMin=[]  SumOutMax=[]  SaturationOutMin=[]  SaturationOutMax=[]  PParamMin=[]  PParamMax=[]  IParamMin=[]  IParamMax=[]  DParamMin=[]  DParamMax=[]  NParamMin=[]  NParamMax=[]  KbParamMin=[]  KbParamMax=[]  KtParamMin=[]  KtParamMax=[]  KbOutMin=[]  KbOutMax=[]  KtOutMin=[]  KtOutMax=[]  IntegratorOutMin=[]  IntegratorOutMax=[]  FilterOutMin=[]  FilterOutMax=[]  SumI1OutMin=[]  SumI1OutMax=[]  SumI2OutMin=[]  SumI2OutMax=[]  SumI3OutMin=[]  SumI3OutMax=[]  SumI4OutMin=[]  SumI4OutMax=[]  SumDOutMin=[]  SumDOutMax=[]  DifferentiatorOutMin=[]  DifferentiatorOutMax=[]  FilterDiffOutCoefMin=[]  FilterDiffOutCoefMax=[]  ReciprocalOutMin=[]  ReciprocalOutMax=[]  SumDenOutMin=[]  SumDenOutMax=[]  SumNumOutMin=[]  SumNumOutMax=[]  DivideOutMin=[]  DivideOutMax=[]  UdiffTsProdOutMin=[]  UdiffTsProdOutMax=[]  NTsProdOutMin=[]  NTsProdOutMax=[]  UintegralTsProdOutMin=[]  UintegralTsProdOutMax=[]  UngainTsProdOutMin=[]  UngainTsProdOutMax=[]  ClampingZeroOutDataTypeStr=Inherit: Inherit via back propagation  ClampingZeroOutMin=[]  ClampingZeroOutMax=[]  FilterDenConstantOutDataTypeStr=Inherit: Inherit via back propagation  FilterDenConstantOutMin=[]  FilterDenConstantOutMax=[]  PCopyOutDataTypeStr=Inherit: Inherit via back propagation  PCopyOutMin=[]  PCopyOutMax=[]  NCopyOutDataTypeStr=Inherit: Inherit via back propagation  NCopyOutMin=[]  NCopyOutMax=[]  IntegratorContinuousStateAttributes=''  IntegratorStateMustResolveToSignalObject=off  IntegratorRTWStateStorageClass=Auto  FilterContinuousStateAttributes=''  FilterStateMustResolveToSignalObject=off  FilterRTWStateStorageClass=Auto  ParallelPVariant=InternalParameters  IdealPVariant=Disabled  IVariant=InternalParameters  DVariant=Disabled  IntegratorVariant=Continuous  SatVariant=Disabled  AWVariant=Passthrough  PCopyVariant=Disabled  TRVariant=Disabled  FdbkBlocksVariant=Forward  IdealPFdbkVariant=Disabled  SatFdbkVariant=Disabled  DerivativeFilterVariant=Disabled  NVariant=Disabled  NCopyVariant=Disabled_SignalSpec  FilterICVariant=Disabled  IntegratorICVariant=InternalICs  ExternalResetVariant=Disabled  TRSumVariant=Passthrough  SumFdbkVariant=Disabled  SumVariant=Sum_PI  TsampFilterVariant=InternalTs  TsampNgainVariant=Passthrough  TsampIntegralVariant=Disabled_SignalSpec  ExternalSaturationOutDataTypeStr=Inherit: Same as second input
  Mux : Mux  Inputs=3
  PWM Generator (2-Level) : spsPWMGenerator2LevelLib/PWM Generator (2-Level)  ModulatorType=Three-phase bridge (6 pulses)  ModulatorMode=Unsynchronized  Fc=fsw  Pc=0  nF=27  MinMax="[ -1  1 ]"  SamplingTechnique=Natural  ModulatingSignals=off  m=0.8  Freq=60  Phase=0  Ts=0  ShowCarrierOutport=off
  Scope : Scope  NumInputPorts=2
  Scope1 : Scope
  Scope2 : Scope  NumInputPorts=2
  Sum : Sum  Inputs=|+-
  Sum1 : Sum  Inputs=-+|
  Sum2 : Sum  Inputs=|++
  Sum3 : Sum  Inputs=-+|
  Sum4 : Sum  Inputs=|++
  Sum5 : Sum  Inputs=++|
  Terminator1 : Terminator
  abc to dq1 : spsabctodq0Lib/abc to dq0  Alignment=90 degrees behind phase A axis
  dq0 to abc : spsdq0toabcLib/dq0 to abc  Alignment=90 degrees behind phase A axis
  wL : Gain  Gain=2*pi*f*L
  PWM : Outport
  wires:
  PWM Generator (2-Level)/1 -> PWM/1
  Id PI Controller/1 -> Scope2/1, Sum2/1
  Gain2/1 -> PWM Generator (2-Level)/1
  Ground/1 -> Mux/3
  wL/1 -> Sum3/1
  Gain/1 -> Sum2/2
  dq0 to abc/1 -> Scope1/1, Gain2/1
  vd_grid/1 -> Sum4/2
  Sum1/1 -> Iq PD Controller/1
  Sum/1 -> Id PI Controller/1
  abc to dq1/1 -> Demux/1
  Sum2/1 -> Sum4/1
  Mux/1 -> dq0 to abc/1
  vq_grid/1 -> Sum5/1
  Sum3/1 -> Sum5/2
  Sum5/1 -> Mux/2
  Demux/1 -> Scope/1, Sum/2, wL/1
  Iq PD Controller/1 -> Scope2/2, Sum3/2
  Sum4/1 -> Mux/1
  Demux/2 -> Sum1/1, Gain/1, Scope/2
  Demux/3 -> Terminator1/1
  Iinv/1 -> abc to dq1/1
  Iq*/1 -> Sum1/2
  id*/1 -> Sum/1
  wt/1 -> abc to dq1/2, dq0 to abc/2

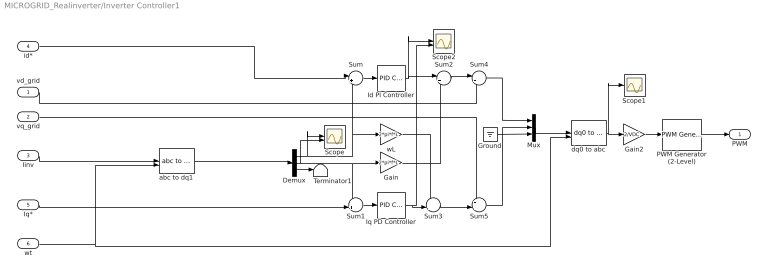
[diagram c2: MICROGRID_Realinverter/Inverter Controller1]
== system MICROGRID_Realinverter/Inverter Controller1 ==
  vd_grid : Inport
  vq_grid : Inport  Port=2
  Iinv : Inport  Port=3
  id* : Inport  Port=4
  Iq* : Inport  Port=5
  wt : Inport  Port=6
  Demux : Demux  Outputs=3
  Gain : Gain  Gain=2*pi*f*L
  Gain2 : Gain  Gain=2/VDC
  Ground : Ground
  Id PI Controller : slpidlib/PID Controller  Controller=PI  Form=Parallel  TimeDomain=Continuous-time  UseExternalTs=off  SampleTime=-1  IntegratorMethod=Forward Euler  FilterMethod=Forward Euler  ControllerParametersSource=internal  P=kp  I=ki  UseKiTs=off  D=0  N=100  UseFilter=on  TunerSelectOption=Transfer Function Based (PID Tuner App)  InitialConditionSource=internal  InitialConditionForIntegrator=0  InitialConditionForFilter=0  DifferentiatorICPrevScaledInput=0  ExternalReset=none  TrackingMode=off  Kt=1  LimitOutput=off  SatLimitsSource=internal  UpperSaturationLimit=inf  LowerSaturationLimit=-inf  LinearizeAsGain=on  AntiWindupMode=none  Kb=1  LimitIntegrator=off  UpperIntegratorSaturationLimit=inf  LowerIntegratorSaturationLimit=-inf  POutMin=[]  POutMax=[]  IOutMin=[]  IOutMax=[]  DOutMin=[]  DOutMax=[]  NOutMin=[]  NOutMax=[]  SumOutMin=[]  SumOutMax=[]  SaturationOutMin=[]  SaturationOutMax=[]  PParamMin=[]  PParamMax=[]  IParamMin=[]  IParamMax=[]  DParamMin=[]  DParamMax=[]  NParamMin=[]  NParamMax=[]  KbParamMin=[]  KbParamMax=[]  KtParamMin=[]  KtParamMax=[]  KbOutMin=[]  KbOutMax=[]  KtOutMin=[]  KtOutMax=[]  IntegratorOutMin=[]  IntegratorOutMax=[]  FilterOutMin=[]  FilterOutMax=[]  SumI1OutMin=[]  SumI1OutMax=[]  SumI2OutMin=[]  SumI2OutMax=[]  SumI3OutMin=[]  SumI3OutMax=[]  SumI4OutMin=[]  SumI4OutMax=[]  SumDOutMin=[]  SumDOutMax=[]  DifferentiatorOutMin=[]  DifferentiatorOutMax=[]  FilterDiffOutCoefMin=[]  FilterDiffOutCoefMax=[]  ReciprocalOutMin=[]  ReciprocalOutMax=[]  SumDenOutMin=[]  SumDenOutMax=[]  SumNumOutMin=[]  SumNumOutMax=[]  DivideOutMin=[]  DivideOutMax=[]  UdiffTsProdOutMin=[]  UdiffTsProdOutMax=[]  NTsProdOutMin=[]  NTsProdOutMax=[]  UintegralTsProdOutMin=[]  UintegralTsProdOutMax=[]  UngainTsProdOutMin=[]  UngainTsProdOutMax=[]  ClampingZeroOutDataTypeStr=Inherit: Inherit via back propagation  ClampingZeroOutMin=[]  ClampingZeroOutMax=[]  FilterDenConstantOutDataTypeStr=Inherit: Inherit via back propagation  FilterDenConstantOutMin=[]  FilterDenConstantOutMax=[]  PCopyOutDataTypeStr=Inherit: Inherit via back propagation  PCopyOutMin=[]  PCopyOutMax=[]  NCopyOutDataTypeStr=Inherit: Inherit via back propagation  NCopyOutMin=[]  NCopyOutMax=[]  IntegratorContinuousStateAttributes=''  IntegratorStateMustResolveToSignalObject=off  IntegratorRTWStateStorageClass=Auto  FilterContinuousStateAttributes=''  FilterStateMustResolveToSignalObject=off  FilterRTWStateStorageClass=Auto  ParallelPVariant=InternalParameters  IdealPVariant=Disabled  IVariant=InternalParameters  DVariant=Disabled  IntegratorVariant=Continuous  SatVariant=Disabled  AWVariant=Passthrough  PCopyVariant=Disabled  TRVariant=Disabled  FdbkBlocksVariant=Forward  IdealPFdbkVariant=Disabled  SatFdbkVariant=Disabled  DerivativeFilterVariant=Disabled  NVariant=Disabled  NCopyVariant=Disabled_SignalSpec  FilterICVariant=Disabled  IntegratorICVariant=InternalICs  ExternalResetVariant=Disabled  TRSumVariant=Passthrough  SumFdbkVariant=Disabled  SumVariant=Sum_PI  TsampFilterVariant=InternalTs  TsampNgainVariant=Passthrough  TsampIntegralVariant=Disabled_SignalSpec  ExternalSaturationOutDataTypeStr=Inherit: Same as second input
  Iq PD Controller : slpidlib/PID Controller  Controller=PI  Form=Parallel  TimeDomain=Continuous-time  UseExternalTs=off  SampleTime=-1  IntegratorMethod=Forward Euler  FilterMethod=Forward Euler  ControllerParametersSource=internal  P=kp  I=ki  UseKiTs=off  D=0  N=100  UseFilter=on  TunerSelectOption=Transfer Function Based (PID Tuner App)  InitialConditionSource=internal  InitialConditionForIntegrator=0  InitialConditionForFilter=0  DifferentiatorICPrevScaledInput=0  ExternalReset=none  TrackingMode=off  Kt=1  LimitOutput=off  SatLimitsSource=internal  UpperSaturationLimit=inf  LowerSaturationLimit=-inf  LinearizeAsGain=on  AntiWindupMode=none  Kb=1  LimitIntegrator=off  UpperIntegratorSaturationLimit=inf  LowerIntegratorSaturationLimit=-inf  POutMin=[]  POutMax=[]  IOutMin=[]  IOutMax=[]  DOutMin=[]  DOutMax=[]  NOutMin=[]  NOutMax=[]  SumOutMin=[]  SumOutMax=[]  SaturationOutMin=[]  SaturationOutMax=[]  PParamMin=[]  PParamMax=[]  IParamMin=[]  IParamMax=[]  DParamMin=[]  DParamMax=[]  NParamMin=[]  NParamMax=[]  KbParamMin=[]  KbParamMax=[]  KtParamMin=[]  KtParamMax=[]  KbOutMin=[]  KbOutMax=[]  KtOutMin=[]  KtOutMax=[]  IntegratorOutMin=[]  IntegratorOutMax=[]  FilterOutMin=[]  FilterOutMax=[]  SumI1OutMin=[]  SumI1OutMax=[]  SumI2OutMin=[]  SumI2OutMax=[]  SumI3OutMin=[]  SumI3OutMax=[]  SumI4OutMin=[]  SumI4OutMax=[]  SumDOutMin=[]  SumDOutMax=[]  DifferentiatorOutMin=[]  DifferentiatorOutMax=[]  FilterDiffOutCoefMin=[]  FilterDiffOutCoefMax=[]  ReciprocalOutMin=[]  ReciprocalOutMax=[]  SumDenOutMin=[]  SumDenOutMax=[]  SumNumOutMin=[]  SumNumOutMax=[]  DivideOutMin=[]  DivideOutMax=[]  UdiffTsProdOutMin=[]  UdiffTsProdOutMax=[]  NTsProdOutMin=[]  NTsProdOutMax=[]  UintegralTsProdOutMin=[]  UintegralTsProdOutMax=[]  UngainTsProdOutMin=[]  UngainTsProdOutMax=[]  ClampingZeroOutDataTypeStr=Inherit: Inherit via back propagation  ClampingZeroOutMin=[]  ClampingZeroOutMax=[]  FilterDenConstantOutDataTypeStr=Inherit: Inherit via back propagation  FilterDenConstantOutMin=[]  FilterDenConstantOutMax=[]  PCopyOutDataTypeStr=Inherit: Inherit via back propagation  PCopyOutMin=[]  PCopyOutMax=[]  NCopyOutDataTypeStr=Inherit: Inherit via back propagation  NCopyOutMin=[]  NCopyOutMax=[]  IntegratorContinuousStateAttributes=''  IntegratorStateMustResolveToSignalObject=off  IntegratorRTWStateStorageClass=Auto  FilterContinuousStateAttributes=''  FilterStateMustResolveToSignalObject=off  FilterRTWStateStorageClass=Auto  ParallelPVariant=InternalParameters  IdealPVariant=Disabled  IVariant=InternalParameters  DVariant=Disabled  IntegratorVariant=Continuous  SatVariant=Disabled  AWVariant=Passthrough  PCopyVariant=Disabled  TRVariant=Disabled  FdbkBlocksVariant=Forward  IdealPFdbkVariant=Disabled  SatFdbkVariant=Disabled  DerivativeFilterVariant=Disabled  NVariant=Disabled  NCopyVariant=Disabled_SignalSpec  FilterICVariant=Disabled  IntegratorICVariant=InternalICs  ExternalResetVariant=Disabled  TRSumVariant=Passthrough  SumFdbkVariant=Disabled  SumVariant=Sum_PI  TsampFilterVariant=InternalTs  TsampNgainVariant=Passthrough  TsampIntegralVariant=Disabled_SignalSpec  ExternalSaturationOutDataTypeStr=Inherit: Same as second input
  Mux : Mux  Inputs=3
  PWM Generator (2-Level) : spsPWMGenerator2LevelLib/PWM Generator (2-Level)  ModulatorType=Three-phase bridge (6 pulses)  ModulatorMode=Unsynchronized  Fc=fsw  Pc=0  nF=27  MinMax="[ -1  1 ]"  SamplingTechnique=Natural  ModulatingSignals=off  m=0.8  Freq=60  Phase=0  Ts=0  ShowCarrierOutport=off
  Scope : Scope  NumInputPorts=2
  Scope1 : Scope
  Scope2 : Scope  NumInputPorts=2
  Sum : Sum  Inputs=|+-
  Sum1 : Sum  Inputs=-+|
  Sum2 : Sum  Inputs=|++
  Sum3 : Sum  Inputs=-+|
  Sum4 : Sum  Inputs=|++
  Sum5 : Sum  Inputs=++|
  Terminator1 : Terminator
  abc to dq1 : spsabctodq0Lib/abc to dq0  Alignment=90 degrees behind phase A axis
  dq0 to abc : spsdq0toabcLib/dq0 to abc  Alignment=90 degrees behind phase A axis
  wL : Gain  Gain=2*pi*f*L
  PWM : Outport
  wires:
  PWM Generator (2-Level)/1 -> PWM/1
  Id PI Controller/1 -> Scope2/1, Sum2/1
  Gain2/1 -> PWM Generator (2-Level)/1
  Ground/1 -> Mux/3
  wL/1 -> Sum3/1
  Gain/1 -> Sum2/2
  dq0 to abc/1 -> Scope1/1, Gain2/1
  vd_grid/1 -> Sum4/2
  Sum1/1 -> Iq PD Controller/1
  Sum/1 -> Id PI Controller/1
  abc to dq1/1 -> Demux/1
  Sum2/1 -> Sum4/1
  Mux/1 -> dq0 to abc/1
  vq_grid/1 -> Sum5/1
  Sum3/1 -> Sum5/2
  Sum5/1 -> Mux/2
  Demux/1 -> Scope/1, Sum/2, wL/1
  Iq PD Controller/1 -> Scope2/2, Sum3/2
  Sum4/1 -> Mux/1
  Demux/2 -> Sum1/1, Gain/1, Scope/2
  Demux/3 -> Terminator1/1
  Iinv/1 -> abc to dq1/1
  Iq*/1 -> Sum1/2
  id*/1 -> Sum/1
  wt/1 -> abc to dq1/2, dq0 to abc/2
